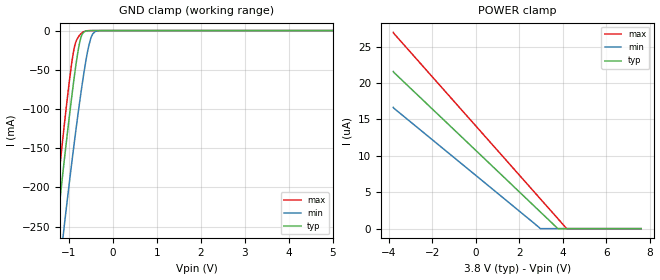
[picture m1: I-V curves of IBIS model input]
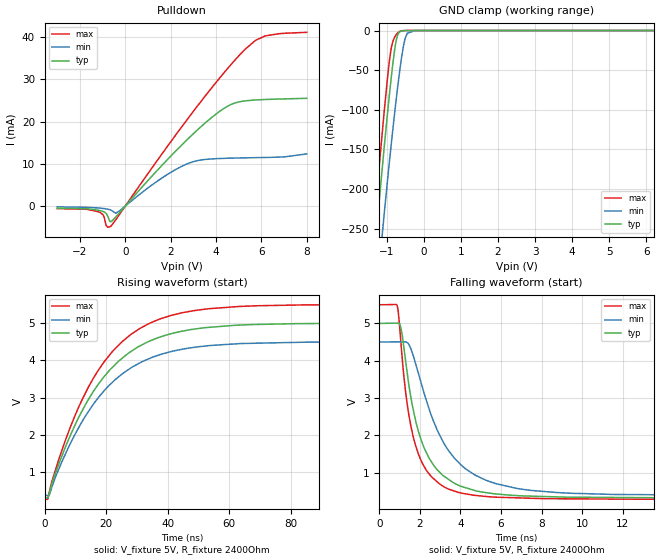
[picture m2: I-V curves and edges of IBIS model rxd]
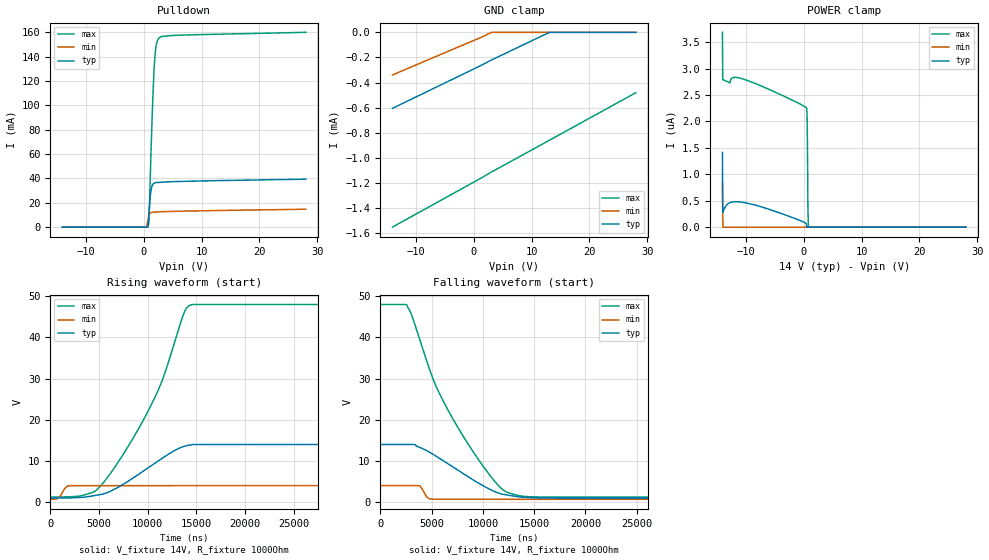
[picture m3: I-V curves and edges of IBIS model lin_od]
|Texas Instruments Incorporated
|TLIN2022-Q1 Fault Protected Dual Local Interconnect Network (LIN) Transceiver
|with Dominant State Timeout
[IBIS Ver]   4.1
[File name]   tlin2022-q1.ibs
[Date]   01/05/2017
[File Rev]   1.0
[Source]
| Texas Instruments Incorporated.
| Analog-eLab Design Center, HPA
| 12500 TI Blvd
| Dallas, TX -75243
[Notes]
| Rev 1.0: 01/05/2017
| - Initial version of the model
| - Model generated from simulations in SPECTRE
| - Model matched to SPICE simulation
| - C_comp although listed in numerical order of value are
|   obtained from varying PVT conditions. For PVT conditions for
|   each specific value refer the buffer description under
|   respective [Model]. IBIS model user is responsible for using
|   appropriate C_comp to simulate for Signal Integrity.
| - Warnings regarding combined Non-monotonicity of various models
|   have been reviewed and considered minor and can be ignored.
| - slow corner of lin_output model correlated for frequencies from 2KHz to 10KHz
[Disclaimer]
| This model is designed as an aid for customers of Texas Instruments.
| TI and its licensors and suppliers make no warranties, either expressed
| or implied, with respect to this  model, including the warranties of
| merchantability or fitness for a particular purpose. The model is
| provided solely on an "as is" basis. The entire risk as to its quality
| and performance is with the customer.
[Copyright]
(C) Copyright 2018 Texas Instruments Incorporated.All rights reserved.
|  Component TLIN2022DRQ1 14-pin SOIC - D package
|  Part # TLIN2022DRQ1
[Component]   TLIN2022DRQ1
[Manufacturer]  TI
[Package]   |14 SOIC - D package
|   typ   min   max
R_pkg   0.1   0.08   0.12
L_pkg   1.0nH   0.8nH   1.2nH
C_pkg   0.2pF   0.16pF   0.24pF
[Pin]  signal_name model_name   R_pin   L_pin   C_pin
1   RXD1   rxd   NA   NA   NA
2   EN1   input   NA   NA   NA
3   TXD1   input   NA   NA   NA
4   RXD2   rxd   NA   NA   NA
5   EN2   input   NA   NA   NA
6   NC   nc   NA   NA   NA
7   TXD2   input   NA   NA   NA
8   GND   gnd   NA   NA   NA
9   LIN2   lin   NA   NA   NA
10   VSUP   power   NA   NA   NA
11   NC   nc   NA   NA   NA
12   NC   nc   NA   NA   NA
13   LIN1   lin   NA   NA   NA
14   NC   nc   NA   NA   NA
|  Component TLIN2022DMTRQ1 14-pin VSON - DMT package
|  Part # TLIN2022DMTRQ1
[Component]   TLIN2022DMTRQ1
[Manufacturer]  TI
[Package]   |14 VSON - DMT package
|   typ   min   max
R_pkg   0   0   0
L_pkg   0   0   0
C_pkg   0   0   0
[Pin]  signal_name model_name   R_pin   L_pin   C_pin
1   RXD1   rxd   NA   NA   NA
2   EN1   input   NA   NA   NA
3   TXD1   input   NA   NA   NA
4   RXD2   rxd   NA   NA   NA
5   EN2   input   NA   NA   NA
6   NC   nc   NA   NA   NA
7   TXD2   input   NA   NA   NA
8   GND   gnd   NA   NA   NA
9   LIN2   lin   NA   NA   NA
10   VSUP   power   NA   NA   NA
11   NC   nc   NA   NA   NA
12   NC   nc   NA   NA   NA
13   LIN1   lin   NA   NA   NA
14   NC   nc   NA   NA   NA
|   Model Selectors
[Model Selector] lin
lin_od   14.0V   digital I/O_open_drain
lin_output   14.0V   digital Output
| Models and submodels in the file (4): input (Input), rxd (Open_sink), lin_od (I/O_open_drain), lin_output (Output)
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|   input Model
[Model]   input
Model_type   Input
Vinl = 0.8
Vinh = 2
|   typ   min   max
C_comp   3.46465E-12   3.07372E-12   4.01486E-12
| Where Nom  PVT is Nominal Process, 3.8V, 27C
|   Fast PVT is Strong Process,  4.2V, -55C
|   Slow PVT is Weak Process,   3V, 165C
[Voltage Range]   3.8   3   4.2
|Junction Temperature
[Temperature Range]   27   165   -55
[Power Clamp Reference]   3.8   3   4.2
[GND Clamp Reference]   0   0   0
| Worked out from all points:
|   GND clamp passes 1 mA (typ) near -0.63 V on its own axis
[GND Clamp]
|   Voltage   I(typ)   I(min)   I(max)
-3.8V     -1.716A    -1.741A    -1.714A
-1.417V   -329.7mA   -408.3mA   -288.7mA
-1.292V   -261.7mA   -342.8mA   -218.9mA
-1.269V   -249.6mA   -331mA     -206.5mA
-1.11V    -167.2mA   -250.8mA   -122.4mA
-904.4mV  -70.09mA   -154.5mA   -29.5mA
-847.4mV  -46.14mA   -129.4mA   -15.27mA
-767.6mV  -18.24mA   -95.69mA   -6.643mA
-665mV    -2.116mA   -55.77mA   -1.406mA
-494mV    -29.94uA   -8.423mA   -15.55uA
-300.2mV  -812.1nA   -88.71uA   -911.7nA
7.6V      0A         0A         0A
[POWER Clamp]
|   Voltage   I(typ)   I(min)   I(max)
-3.8V     21.6uA     16.67uA    26.97uA
2.96V     2.302uA    13.73nA    4.1uA
3.758V    23.08nA    0A         1.408uA
4.169V    0A         0A         15.11nA
7.6V      0A         0A         0A
|   rxd Model
[Model]   rxd
Model_type   Open_sink
Polarity   Non-Inverting
Vmeas = 2.5
Vref = 5
Cref = 2pF
Rref = 2400
|   typ   min   max
C_comp   3.72956E-12   3.27827E-12   4.2623E-12
| Where Nom  PVT is Nominal Process, 5V, 27C
|   Fast PVT is Strong Process,  5.5V, -55C
|   Slow PVT is Weak Process,   4.5V, 165C
[Voltage Range]   5   4.5   5.5
|Junction Temperature
[Temperature Range]   27   165   -55
[Pullup Reference]   5   4.5   5.5
[Pulldown Reference]   0   0   -0
[Power Clamp Reference]   5   4.5   5.5
[GND Clamp Reference]   0   0   0
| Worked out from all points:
|   slope of the pulldown table from 0 to 0.75 V, typ, clamps not added: 164 ohm
|   GND clamp passes 1 mA (typ) near -0.63 V on its own axis
|   falling waveform, V_fixture 5V, R_fixture 2400Ohm: 20-80 % time 1.33ns typ, 2.1ns min, 989ps max; typ from 5 V to 0.318 V
|   rising waveform, V_fixture 5V, R_fixture 2400Ohm: 20-80 % time 20.5ns typ, 20.7ns min, 20.1ns max; typ from 0.318 V to 5 V
[Pulldown]
|   Voltage   I(typ)   I(min)   I(max)
-3V       -478.7uA   -191.2uA   -603.9uA
-1.174V   -992.2uA   -450.9uA   -1.367mA
-965mV    -1.321mA   -581.3uA   -2.223mA
-844mV    -1.756mA   -677uA     -4.594mA
-646mV    -3.719mA   -938.5uA   -4.804mA
-426mV    -2.622mA   -1.694mA   -3.306mA
1.51V     9.031mA    6.263mA    11.55mA
2.841V    16.32mA    10.23mA    21.3mA
4.381V    23.25mA    11.31mA    31.77mA
5.283V    24.93mA    11.43mA    37.15mA
6.174V    25.26mA    11.51mA    40.34mA
8V        25.54mA    12.36mA    41.18mA
[GND Clamp]
|   Voltage   I(typ)   I(min)   I(max)
-3V       -1.245A    -1.286A    -1.23A
-1.559V   -408.7mA   -484.2mA   -369.9mA
-1.284V   -257.7mA   -339mA     -214.7mA
-1.086V   -155.7mA   -239.7mA   -110.7mA
-910mV    -72.76mA   -157.3mA   -31.65mA
-833mV    -40.68mA   -123.5mA   -13.39mA
-767mV    -18.25mA   -95.75mA   -6.8mA
-635mV    -1.061mA   -45.43mA   -766.8uA
-536mV    -90.64uA   -16.53mA   -55.21uA
-448mV    -8.124uA   -3.48mA    -2.688uA
-239mV    0A         -18.54uA   0A
8V        0A         0A         0A
[POWER Clamp]
|   Voltage   I(typ)   I(min)   I(max)
-3V       0A         0A         0A
0V        0A         0A         0A
8V        0A         0A         0A
[Ramp]
R_load = 2400
|   typ   min   max
dV/dt_r   2.80934/2.05464e-08   2.46843/2.06734e-08   3.13188/2.01086e-08
dV/dt_f   2.80935/1.32286e-09   2.46843/2.098e-09   3.13188/9.89047e-10
[Falling Waveform]
V_fixture = 5V
V_fixture_min = 4.5V
V_fixture_max = 5.5V
R_fixture = 2400Ohm
C_fixture = 0F
|   Time   V(typ)   V(min)   V(max)
0s        5V         4.5V       5.5V
877.3ps   5.007V     4.505V     5.486V
1.073ns   4.858V     4.506V     4.422V
1.389ns   3.611V     4.479V     2.779V
2.02ns    1.942V     3.48V      1.367V
2.871ns   1.064V     2.115V     740.3mV
4.079ns   620.7mV    1.177V     442.5mV
5.756ns   424.7mV    699.4mV    337.5mV
9.477ns   337.3mV    442.6mV    293.3mV
40ns      317.8mV    385.9mV    280.2mV
[Rising Waveform]
V_fixture = 5V
V_fixture_min = 4.5V
V_fixture_max = 5.5V
R_fixture = 2400Ohm
C_fixture = 0F
|   Time   V(typ)   V(min)   V(max)
0s        317.8mV    385.9mV    280.2mV
943.3ps   319.6mV    384.8mV    279.9mV
1.502ns   449.3mV    398.4mV    480.9mV
6.576ns   1.653V     1.468V     1.83V
11.47ns   2.545V     2.266V     2.829V
15.68ns   3.152V     2.812V     3.505V
21.94ns   3.811V     3.409V     4.233V
34.19ns   4.521V     4.058V     5V
53.07ns   4.885V     4.395V     5.385V
600ns     5V         4.5V       5.5V
|   lin_od Model
[Model]   lin_od
Model_type   I/O_open_drain
Polarity   Non-Inverting
Enable   Active-High
Vinl = 5.6
Vinh = 8.4
Vmeas = 7
Vref = 14
Cref = 2pF
Rref = 1000
|   typ   min   max
C_comp   3.52891E-11   2.76465E-11   3.67824E-11
[Model spec]
|subparameter
Vinl   5.6   1.6   19.2
Vinh   8.4   2.4   28.8
| Where Nom  PVT is Nominal Process, 14V, 27C
|   Fast PVT is Strong Process,  48V, -55C
|   Slow PVT is Weak Process,   4V, 165C
[Voltage Range]   14   4   48
|Junction Temperature
[Temperature Range]   27   165   -55
[Pullup Reference]   14   4   48
[Pulldown Reference]   0   0   -0
[Power Clamp Reference]   14   4   48
[GND Clamp Reference]   0   0   0
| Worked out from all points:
|   slope of the pulldown table from 0 to 2.1 V, typ, clamps not added: 57.4 ohm
|   falling waveform, V_fixture 14V, R_fixture 1000Ohm: 20-80 % time 5.03us typ, 473ns min, 5.55us max; typ from 14 V to 0.965 V
|   rising waveform, V_fixture 14V, R_fixture 1000Ohm: 20-80 % time 5.04us typ, 524ns min, 5.53us max; typ from 0.965 V to 14 V
[Pulldown]
|   Voltage   I(typ)   I(min)   I(max)
-14V      1.34pA     608.3pA    22.4pA
238mV     339.9nA    1.556uA    263.8nA
742mV     727.2uA    5.435mA    358.5uA
868mV     6.608mA    8.41mA     2.099mA
952mV     12.48mA    9.825mA    8.962mA
1.204V    27.16mA    11.68mA    48.57mA
1.498V    34.3mA     12.15mA    92.74mA
1.708V    35.7mA     12.27mA    118.5mA
1.876V    36.2mA     12.33mA    134mA
2.212V    36.71mA    12.44mA    149.9mA
2.8V      36.79mA    12.58mA    155.7mA
28V       39.37mA    14.71mA    159.9mA
[GND Clamp]
|   Voltage   I(typ)   I(min)   I(max)
-14V      -605.9uA   -340uA     -1.551mA
3.178V    -218uA     -283nA     -1.109mA
13.17V    -67.71nA   0A         -856.9uA
28V       0A         0A         -480.5uA
[POWER Clamp]
|   Voltage   I(typ)   I(min)   I(max)
-14V      1.413uA    828.1nA    3.686uA
-13.96V   277.9nA    414nA      2.791uA
-13.92V   290.9nA    0A         2.789uA
-12.99V   446.6nA    0A         2.745uA
-10.81V   474.6nA    0A         2.814uA
490mV     55.91nA    0A         2.26uA
574mV     13.2nA     0A         2.195uA
616mV     0A         0A         2.031uA
658mV     0A         0A         1.671uA
742mV     0A         0A         443.9nA
826mV     0A         0A         0A
28V       0A         0A         0A
[Ramp]
R_load = 1000
|   typ   min   max
dV/dt_r   7.82062/5.00911e-06   2/5.10843e-07   28.078/5.5292e-06
dV/dt_f   7.82061/5.0116e-06   2.00001/4.70726e-07   28.0779/5.54791e-06
[Falling Waveform]
V_fixture = 14V
V_fixture_min = 4V
V_fixture_max = 48V
R_fixture = 1000Ohm
C_fixture = 0F
|   Time   V(typ)   V(min)   V(max)
0s        14V        4V         48V
2.59us    14V        4V         47.89V
3.81us    13.32V     3.962V     39.78V
4.592us   12.41V     1.111V     33.79V
5.194us   11.55V     675.9mV    29.61V
6.494us   9.475V     675.6mV    22.85V
9.958us   4.055V     674.9mV    8.945V
12.38us   1.723V     674.4mV    2.365V
15.99us   1.005V     673.6mV    1.217V
50us      964.9mV    666.4mV    1.201V
[Rising Waveform]
V_fixture = 14V
V_fixture_min = 4V
V_fixture_max = 48V
R_fixture = 1000Ohm
C_fixture = 0F
|   Time   V(typ)   V(min)   V(max)
0s        964.9mV    666.4mV    1.201V
802.7ns   988.3mV    930.1mV    1.229V
1.888us   1.02V      3.963V     1.275V
4.294us   1.481V     3.991V     2.313V
6.094us   2.531V     3.991V     6.7V
10.76us   9.48V      3.992V     25.56V
11.77us   11.08V     3.992V     31.42V
13.67us   13.5V      3.992V     45.6V
14.34us   13.84V     3.993V     47.84V
50us      14V        4V         48V
